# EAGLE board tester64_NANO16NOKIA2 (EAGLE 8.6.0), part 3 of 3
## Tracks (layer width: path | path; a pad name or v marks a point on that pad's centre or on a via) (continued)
PB6_7 (continued)
  Top 0.305: U7.7 191.38,120 192.5,121.12 208.62,121.12 216,128.5 216,134.62 211,139.62 170.38,139.62 165.5,134.75 J2.47 164.38,134.75 163.12,133.5 157.38,133.5 155.62,135.25 154.3,135.25 J4.47 154.08,135.12 153.38,135.12 153.38,135 152.38,134 144.83,134 J6.47
PB6_8
  Top 0.305: 191.62,146.78 191.62,147.25 192.88,148.5 212.5,148.5 212.62,148.62
  Top 0.406: 212.62,148.62 216,152 216,159.38 212,163.38 174.62,163.38 166.32,155.07 J2.63 | 191.62,146.78 U8.7
PB7_1
  Bottom 0.305: U2.8 31.51,53.24 28,56.75 28,64.25 29.62,65.88 35.88,65.88 37.25,64.5 41.8,64.5 RN2.8
PB7_2
  Bottom 0.305: U3.8 30.88,80.74 28,83.62 28,91.88 30,93.88 36.12,93.88 38.75,91.25 42.92,91.25 RN4.8
PB7_3
  Bottom 0.305: U1.8 36.14,112.61 32.5,116.25 32.5,124.25 34,125.75 39.5,125.75 42.25,123 45.8,123 RN6.8
PB7_4
  Bottom 0.305: 36.74,139.5 U4.8 35.39,139.62 32.5,142.5 32.5,152.25 34.5,154.25 40,154.25 44.7,149.55 RN8.8
PB7_5
  Top 0.305: U5.8 192.88,65.51 193.38,66 193.38,66.12 196,68.75 212.25,68.75 216.88,73.38 216.88,83.25 213.25,86.88 183.62,86.88 175.12,95.38 163.37,95.38 J2.16 161.97,94.25 161.38,94.25 159.88,95.75 153.25,95.75 152.16,94.66 J4.16
  Top 0.406: C24.1 U5.8 | J10.16 120.41,93.71 121.62,92.5 123.38,92.5 124.62,93.75 130.33,93.75 J8.16 131.35,93.9 132.75,92.5 141.43,92.5 J6.16 | J13.16 124.46,157.71 125.75,159 130.5,159 131.72,157.78 J15.16 139.4,157.78 140.25,158.62 141.38,158.62 142.76,157.24 J17.16
  Bottom 0.305: RN10.8 139.68,90.75 J6.16 141.61,92.73 142.75,93.88 150.25,93.88 151.12,94.75 151.62,94.75 J4.16
  Bottom 0.406: J13.16 121.41,157.71 120.25,158.88 119.25,158.88 117.88,157.5 117.88,95.25 119.12,94 119.81,94 J10.16
PB7_6
  Top 0.305: U6.8 192.88,93.66 192.88,94.5 193.38,95 213.38,95 216.88,98.5 216.88,109.12 213.75,112.25 168.62,112.25 165.12,115.75 164,115.75 162.68,114.43 J2.32 157.07,114.43 155.12,116.38 153.11,116.38 J4.32
  Top 0.406: C40.1 193,93.53 U6.8 | J10.32 120.1,113.89 121.25,112.75 123.5,112.75 124.75,114 130.26,114 J8.32 130.48,114.02 130.98,114.02 132,113 J6.32
  Bottom 0.305: RN12.8 173.05,111.95 169.38,115.62 163.3,115.62 J2.32
  Bottom 0.406: J6.32 142.25,113 143.5,114.25 150.12,114.25 150.88,115 151.69,115 J4.32
PB7_7
  Top 0.305: 163,134.75 164.25,136 165.75,136 170.12,140.38 211,140.38 216.75,134.62 216.75,128.12 209.5,120.88 209.38,120.88 209.12,120.62 193,120.62 192.62,120.25 U7.8 | J2.48 157.25,134.75 155.5,136.5 152.92,136.5 J4.48 151.04,134.62 142.88,134.62 141.61,133.36 J6.48
  Top 0.406: J2.48 163,134.75
PB7_8
  Top 0.305: 213.25,148 193.25,148 192.76,147.51 U8.8
  Top 0.406: J2.64 162.12,155.09 162.12,155.25 163.5,156.62 166.62,156.62 174,164 212.38,164 216.75,159.62 216.75,151.62 213.75,148.62 213.75,148.5 213.25,148
RST.1
  Bottom 0.61: DIS1.J1.1 190.75,15.58 R136.1
SCE.1
  Bottom 0.61: DIS1.J1.2 193.29,14.79 196.5,18 196.5,18.83 R137.1
SCK.1
  Bottom 0.61: DIS1.J1.5 200.91,15.24 R140.1
SCL  (via drill 0.7, 0.7 pad 0.25)
  Top 0.406: 198.12,144.12 211.38,144.12 v211.62,143.88 | v39.25,134.5 v19.62,134.5
  Top 0.61: U8.12 197.84,144.41 198.12,144.12 | R1.1 202,41.08 ARD1.J2.7 199.92,39 192.38,39 190.38,37 190.38,23.25 v190.25,23.12
  Bottom 0.406: 211.62,58.75 211.62,42.62 210.75,41.75 210.75,39.75 209.5,38.5 203.5,38.5 202,40 202,40.66 ARD1.J2.7 202,41.08 | 211.62,58.75 v211.62,90.62 211.62,100.86 212.22,101.45 212.22,105.26 211.46,106.02 211.46,115.96 211.62,116.12 | 211.62,116.12 211.62,115.88 | v211.62,143.88 211.62,116.12 | U4.12 39.22,134.53 v39.25,134.5 | SW7.5 205.59,60.91 207.62,58.88 211.5,58.88 211.62,58.75 | 187.12,10.88 187,10.88
  Bottom 0.61: v19.62,134.5 19.62,31.5 | 19.62,31.5 19.62,31 | 187.12,10.88 187.12,11.25 | 187.12,11.25 187.12,20 v190.25,23.12 | 187.12,11.25 187.25,11.12 187.25,9 179.75,1.5 42,1.5 19.75,23.75 19.75,31.38 19.62,31.5
SCL1  (via drill 0.7)
  Top 0.305: 198,93 198,93.61 U6.12
  Top 0.406: 222.62,23.25 211.88,12.5 211.88,6.88 210.25,5.25 177.88,5.25 177.38,5.75 v173.75,5.75
  Top 0.5: U5.12 197.97,66.97 v198,67 | v198,91.75 198,93 | U7.12 197.72,117.28 v197.75,117.25 | v35.62,85.38 35.62,86 37.88,88.25 37.88,106.5 v39,107.62 | v34,75.75 34.62,75.75 35.38,75 35.38,73.25 33.62,71.5 33.62,49.5 v34.62,48.5 35.12,48 v40.38,48 | 222.62,41.62 222.62,23.25 | v49.12,29.75 v37.38,29.75
  Top 0.61: U5.12 197.97,61.53 203.25,56.25 205.54,56.25 | 205.54,56.25 205.54,55.95 207.62,53.88 210.12,53.88 221.25,42.75 221.5,42.75 222.62,41.62 | 205.54,56.25 SW7.4
  Bottom 0.406: 39.25,10.12 39.38,10.12 43.75,5.75 v173.75,5.75
  Bottom 0.5: v198,67 v198,91.75 197.75,92 v197.75,117.25 | U2.12 34.28,48.16 v34.62,48.5 | U3.12 32.32,75.75 v34,75.75 34.75,75.75 35.62,76.62 v35.62,85.38 | v39,107.62 36.95,107.62 U1.12 | v37.38,29.75 37.12,39.38 40.5,42.75 40.5,47.88 v40.38,48 | 39.25,10.12 39.25,20 v49.12,29.75
SCL2
  Top 0.406: SW7.6 205.59,65.72 207.75,67.88 212.62,67.88 217.5,72.75 217.5,80.15 J22.6
SDA  (via drill 0.7, 0.7 pad 0.25)
  Top 0.406: U8.13 199.11,145.51 199.75,144.88 212.62,144.88 v213.62,143.88 | v213.62,63 211.41,63 SW7.2 | v20.75,133.25 v39,133.25
  Top 0.5: 190.25,40 190.25,42.5
  Top 0.61: ARD1.J2.8 R2.1 199.2,44.25 192,44.25 190.25,42.5 | v187.75,23.12 187.75,37.5 190.25,40
  Bottom 0.406: v213.62,143.88 213.62,90.75 v213.5,90.62 v213.62,63 213.62,42.62 213.25,42.25 213.25,38.25 212.25,37.25 201.5,37.25 199.25,39.5 ARD1.J2.8 | U4.13 38.98,133.26 v39,133.25
  Bottom 0.61: v20.75,133.25 20.75,24.25 42.5,2.5 178.5,2.5 185.75,9.75 185.75,21.12 v187.75,23.12
SDA1  (via drill 0.7)
  Top 0.406: v176.25,4.75 177.25,3.75 210,3.75 210.06,3.69
  Top 0.5: U6.13 199.24,92.02 v199.5,91.75 | v199.75,67 199.25,66.5 199.25,64.78 U5.13 | U7.13 198.99,117.64 v199.38,117.25 | 32.88,47 32.88,46.38 33.75,45.5 46.88,45.5 v48.62,47.25 | 32.88,47 32.88,73.5 v34.12,74.38 | v37,85.38 37.12,85.38 38.88,87.12 38.88,105.38 v39.62,106.12 | 33,46.88 32.88,47 | SW7.1 223.5,42.2 223.5,22.25 212.75,11.5 212.75,6.38 210.06,3.69
  Top 0.61: U5.13 199.24,62.77 203.5,58.5 207.25,58.5 208.88,56.88 208.88,56.83 SW7.1 | 33,46.88 34.22,46.88 v34.23,46.89
  Bottom 0.406: 38.25,20.75 38.25,10.25 43.5,5 172.75,5 173,4.75 v176.25,4.75
  Bottom 0.5: v199.75,67 199,67.75 199,90 199.5,90.5 v199.5,91.75 199.24,92.02 199.24,92.88 198.62,93.48 198.62,116.12 199.38,116.88 v199.38,117.25 | v37,85.38 37,76.38 35.02,74.39 34,74.39 33.98,74.38 v34.12,74.38 32.62,74.38 32.61,74.39 U3.13 | v39.62,106.12 39.25,106.12 39.12,106.25 36.87,106.25 U1.13 | v48.62,47.25 48.62,31.12 38.25,20.75
  Bottom 0.61: U2.13 v34.23,46.89
SDA2
  Top 0.406: J22.5 223.75,80.4 223.75,69.88 220.81,66.94 219.57,65.7 SW7.3

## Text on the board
tPlace: 1 | 1 | +5V | 1 2 3 | 1 2 3 | 4 | 5 | 6 | 7 | 8 | 9 | 10 | 11 | 12 | 13 | 14 | 15 | 16 | 17 | 18 | 19 | 20 | 21 | 22 | 23 | 24 | 25 | 26 | 27 | 28 | 29 | 30 | 31 | 32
